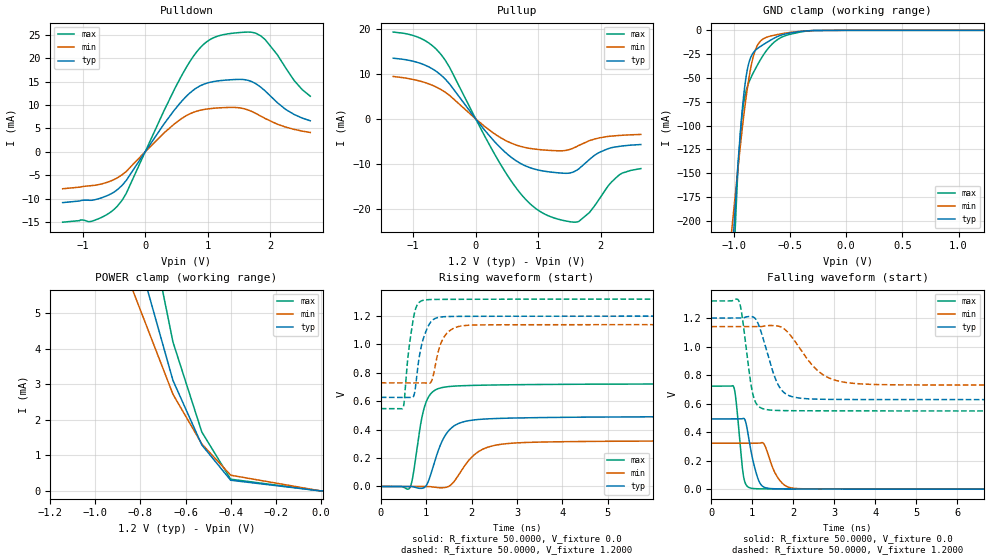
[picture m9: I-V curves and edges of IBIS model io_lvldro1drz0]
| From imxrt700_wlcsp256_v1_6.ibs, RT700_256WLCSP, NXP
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[Model] io_lvldro1drz0
|   Model io_lvldro1drz0
| This model was characterised for following simulation conditions:
| External (pad) voltage:
|   - Typ: 1.2V,   - Min: 1.14V,   - Max: 1.32V
| Library cells for typ/min/max conditions are connected as defined below:
|  ipp_io - External Pad
|  ipp_do - Core Input
|  ipp_obe - Output Buffer Enable
|  config1v21v8 - vdd
|  drive0 - gnde
|  drive1 - vdd
|  gnd - gnd
|  gnde - gnde
|  ncgather - NC
|  vdd - vdd
|  vdde1v8 - vdde1v8
| All other pins connected to ground
Model_type I/O
Polarity   Non-Inverting
Enable   Active-Low
Vinl =   0.3600V
Vinh =   0.8400V
Vmeas =  0.6000V
Cref =   30.0000pF
Rref =   1.0000M
Vref =   1.2000V
C_comp   2.6169pF   2.5664pF   2.7108pF
|C_comp_pullup   1.3450pF   1.4031pF   1.2862pF
|C_comp_pulldown   0.0F   0.0F   0.0F
[Model Spec]
| variable   typ   min   max
Vinh   0.8400V   NA   NA
Vinl   0.3600V   NA   NA
Vref   1.8000V   1.8000V   1.8000V
Cref   30.0000pF   30.0000pF   30.0000pF
Rref   1.0000M   1.0000M   1.0000M
[Temperature Range]   25.0000   0.1250k   -40.0000
[Voltage Range]   1.2000V   1.1400V   1.3200V
[Pullup Reference]   1.2000V   1.1400V   1.3200V
[Pulldown Reference]   0.0V   0.0V   0.0V
[POWER Clamp Reference]   1.2000V   1.1400V   1.3200V
[GND Clamp Reference]   0.0V   0.0V   0.0V
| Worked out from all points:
|   slope of the pulldown table from 0 to 0.18 V, typ, clamps not added: 50.6 ohm
|   slope of the pullup table from 0 to 0.18 V, typ, clamps not added: 57.8 ohm
|   GND clamp passes 1 mA (typ) near -0.39 V on its own axis
|   POWER clamp passes 1 mA (typ) near -0.49 V on its own axis
|   rising waveform, R_fixture 50.0000, V_fixture 0.0: 20-80 % time 384ps typ, 539ps min, 237ps max; typ from 0 V to 0.493 V
|   rising waveform, R_fixture 50.0000, V_fixture 1.2000: 20-80 % time 205ps typ, 227ps min, 166ps max; typ from 0.628 V to 1.2 V
|   falling waveform, R_fixture 50.0000, V_fixture 0.0: 20-80 % time 217ps typ, 294ps min, 140ps max; typ from 0.493 V to 0 V
|   falling waveform, R_fixture 50.0000, V_fixture 1.2000: 20-80 % time 380ps typ, 693ps min, 212ps max; typ from 1.2 V to 0.628 V
[Pulldown]
|Voltage   I(typ)   I(min)   I(max)
-1.32V    -10.88mA   -7.913mA   -15.06mA
-856mV    -10.37mA   -7.241mA   -14.85mA
-448mV    -8.145mA   -5.601mA   -11.68mA
-304mV    -6.16mA    -4.218mA   -8.926mA
296mV     5.851mA    3.961mA    8.642mA
632mV     11.51mA    7.521mA    17.46mA
856mV     13.93mA    8.797mA    21.89mA
1.064V    14.93mA    9.261mA    24.19mA
1.568V    15.45mA    9.245mA    25.55mA
1.84V     13.89mA    7.686mA    24.84mA
2.256V    8.976mA    5.239mA    17.73mA
2.64V     6.622mA    4.125mA    11.88mA
[Pullup]
|Voltage   I(typ)   I(min)   I(max)
-1.32V    13.55mA    9.474mA    19.38mA
-880mV    12.38mA    8.406mA    17.98mA
-560mV    9.836mA    6.583mA    14.46mA
-416mV    7.767mA    5.226mA    11.45mA
488mV     -7.632mA   -4.876mA   -12.18mA
800mV     -10.5mA    -6.394mA   -17.97mA
1.088V    -11.63mA   -6.922mA   -21.12mA
1.464V    -12.12mA   -6.953mA   -22.82mA
1.648V    -11.13mA   -5.911mA   -22.86mA
1.952V    -7.646mA   -4.304mA   -18.35mA
2.304V    -6.102mA   -3.674mA   -12.39mA
2.64V     -5.703mA   -3.453mA   -11.07mA
[GND_clamp]
|Voltage   I(typ)   I(min)   I(max)
-1.32V    -824mA     -526.2mA   -1.227A
-1.032V   -269.6mA   -225.5mA   -323.8mA
-968mV    -148.5mA   -150.4mA   -156.4mA
-936mV    -98.26mA   -114.7mA   -100.6mA
-920mV    -77.35mA   -98.01mA   -82.61mA
-880mV    -41.26mA   -61.23mA   -59.25mA
-856mV    -30.33mA   -43.55mA   -51.86mA
-816mV    -21.94mA   -23.19mA   -42.16mA
-744mV    -15.43mA   -9.413mA   -27.16mA
-584mV    -5.259mA   -3.813mA   -7.801mA
-352mV    -567.9uA   -545.2uA   -812.4uA
1.224V    19.17nA    663.1nA    12.5nA
[POWER_clamp]
|Voltage   I(typ)   I(min)   I(max)
-1.32V    20.02mA    15.02mA    27.66mA
-1.016V   11.22mA    8.62mA     15.53mA
-656mV    3.107mA    2.718mA    4.187mA
-528mV    1.294mA    1.321mA    1.657mA
-400mV    300uA      441.9uA    330.4uA
0V        17.28nA    129.7nA    13.53nA
8mV       16.9nA     117.4nA    13.43nA
[Ramp]
| variable   typ   min   max
dV/dt_r  0.2956/0.3845n   0.1933/0.5381n   0.4336/0.2366n
dV/dt_f  0.3434/0.3799n   0.2461/0.6922n   0.4630/0.2116n
R_load = 50.0000
[Rising Waveform]
R_fixture= 50.0000
V_fixture= 0.0
V_fixture_min= 0.0
V_fixture_max= 0.0
|time   V(typ)   V(min)   V(max)
0s        22.77nV    1.412uV    2.438nV
633.4ps   -4.577uV   610.3nV    -11.9mV
708.5ps   -2.09mV    1.765uV    74.56mV
903.4ps   -13mV      4.359uV    483.7mV
1.038ns   29.97mV    214.9uV    623.5mV
1.402ns   351.3mV    -7.751mV   699.9mV
1.802ns   453.7mV    125.2mV    709.8mV
2.458ns   477.7mV    285.9mV    714.7mV
4.081ns   487.2mV    315.7mV    719.6mV
60ns      492.6mV    322.2mV    722.6mV
[Rising Waveform]
R_fixture= 50.0000
V_fixture= 1.2000
V_fixture_min= 1.1400
V_fixture_max= 1.3200
|time   V(typ)   V(min)   V(max)
0s        627.7mV    729.8mV    548.3mV
492.1ps   627.7mV    729.8mV    556.5mV
606.2ps   627.7mV    729.8mV    936.9mV
714.8ps   631mV      729.8mV    1.179V
891.6ps   987.9mV    729.8mV    1.307V
1.084ns   1.151V     728.4mV    1.317V
1.3ns     1.193V     987.5mV    1.318V
1.434ns   1.196V     1.071V     1.318V
2.119ns   1.199V     1.137V     1.319V
60ns      1.2V       1.14V      1.32V
[Falling Waveform]
R_fixture= 50.0000
V_fixture= 0.0
V_fixture_min= 0.0
V_fixture_max= 0.0
|time   V(typ)   V(min)   V(max)
0s        492.6mV    322.2mV    722.6mV
544.4ps   492.6mV    322.2mV    718.4mV
602.2ps   492.6mV    322.2mV    622.6mV
749.3ps   492.8mV    322.2mV    170.8mV
798.9ps   495.3mV    322.2mV    70.11mV
1.094ns   113.7mV    322.1mV    3.134mV
1.288ns   13.9mV     315.7mV    2.026mV
1.724ns   1.763mV    43.78mV    1.503mV
2.279ns   1.062mV    2.274mV    1.156mV
60ns      274.3nV    3.817uV    18.29nV
[Falling Waveform]
R_fixture= 50.0000
V_fixture= 1.2000
V_fixture_min= 1.1400
V_fixture_max= 1.3200
|time   V(typ)   V(min)   V(max)
0s        1.2V       1.14V      1.32V
664.6ps   1.2V       1.14V      1.324V
738.6ps   1.2V       1.14V      1.239V
949.2ps   1.211V     1.14V      768.4mV
1.049ns   1.203V     1.14V      629.7mV
1.57ns    770.2mV    1.147V     552.4mV
1.904ns   655.1mV    1.088V     550.4mV
2.733ns   630.2mV    801.1mV    549.4mV
3.978ns   628.5mV    734.2mV    548.9mV
60ns      627.7mV    729.8mV    548.3mV
